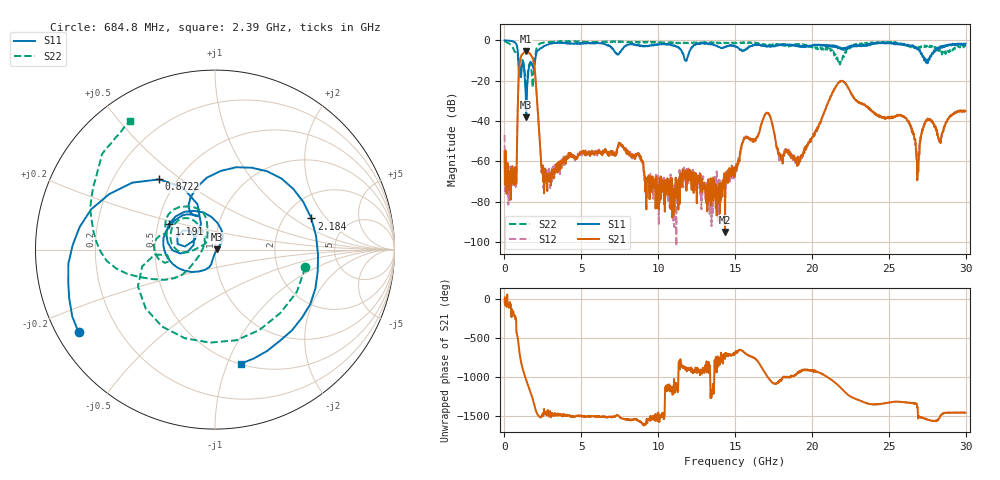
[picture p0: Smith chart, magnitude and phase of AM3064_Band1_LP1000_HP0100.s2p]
# Hz S DB R 50.0
!freq dBS11 angS11 dBS21 angS21 dBS12 angS12 dBS22 angS22
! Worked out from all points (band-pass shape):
!   1600 points, 10 MHz to 29.98 GHz, reference 50 ohm
!   highest |S21| = -5.42 dB at 1.397 GHz (marker M1); lowest = -95.1 dB at 14.35 GHz (marker M2)
!   |S21| within 3 dB of the highest: 1.059 GHz to 1.818 GHz (758.9 MHz wide, 52.7 % of centre)
!   lowest |S11| = -38.2 dB at 1.416 GHz (marker M3), VSWR 1.02, Z = 51.2 + j0.0723 ohm
!   |S11| at or under -10 dB: 902 MHz to 1.995 GHz (1.093 GHz wide, 75.5 % of centre); 27.39161 GHz to 27.46031 GHz (68.7 MHz wide, 0.25 % of centre); 27.48976 GHz to 27.56436 GHz (74.6 MHz wide, 0.271 % of centre)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
!   |S22| runs from -24.0 to -0.3 dB; largest |S21 - S12| = 0.0069
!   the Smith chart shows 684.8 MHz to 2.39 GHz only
!   S11 on the Smith chart (normalised r, x): 684.8 MHz: 0.06, -0.28; 872.2 MHz: 0.40, +0.42; 1.191 GHz: 0.57, +0.18; 2.184 GHz: 2.78, +1.42; 2.39 GHz: 0.51, -1.12
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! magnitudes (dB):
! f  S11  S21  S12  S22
! 10 MHz  -0.1  -55.2  -46.9  -0.3
! 684.8 MHz  -1.0  -62.9  -65.8  -5.8
! 872.2 MHz  -6.0  -31.1  -31.1  -7.6
! 1.191 GHz  -10.7  -6.7  -6.6  -9.8
! 1.397 GHz  -30.0  -5.4  -5.4  -23.6
! 1.416 GHz  -38.2  -5.4  -5.4  -24.0
! 1.866 GHz  -13.4  -9.5  -9.5  -21.1
! 2.184 GHz  -5.0  -36.7  -36.8  -2.5
! 2.39 GHz  -3.7  -62.7  -59.8  -1.3
! 5.015 GHz  -1.5  -56.0  -55.8  -0.6
! 7.582 GHz  -5.4  -51.7  -52.3  -0.5
! 10 GHz  -2.0  -72.1  -70.9  -0.9
! 14.35 GHz  -3.4  -95.1  -69.7  -1.2
! 15 GHz  -3.1  -66.4  -62.7  -1.4
! 17.05 GHz  -2.8  -36.1  -35.8  -2.5
! 17.95 GHz  -2.4  -57.7  -57.4  -2.0
! 19.99 GHz  -2.8  -48.6  -48.7  -3.1
! 21.9 GHz  -4.3  -20.2  -20.0  -9.5
! 25 GHz  -1.1  -38.7  -38.3  -1.1
! 26.89 GHz  -4.2  -62.1  -63.5  -3.5
! 27.51 GHz  -10.8  -39.8  -39.3  -3.4
! 29.98 GHz  -1.7  -35.0  -35.4  -3.1
